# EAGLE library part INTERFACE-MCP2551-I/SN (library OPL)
High speed CAN transceiver
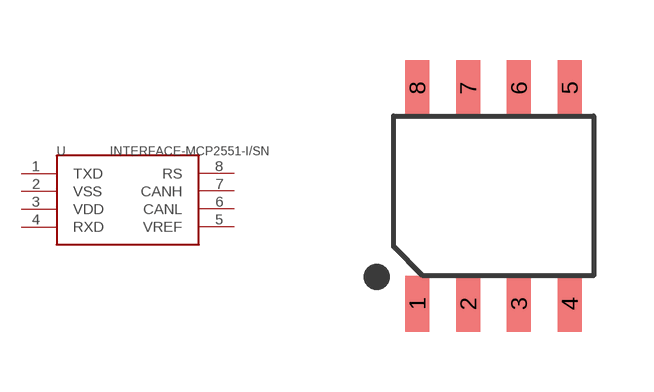
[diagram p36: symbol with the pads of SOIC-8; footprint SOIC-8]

Designator prefix U

## INTERFACE-MCP2551-I/SN-310070024  [SOIC-8]
1  TXD
2  VSS
3  VDD
4  RXD
5  VREF
6  CANL
7  CANH
8  RS

## Footprint SOIC-8 (pad centres in mm)
smd 0.6 x 1.4: 1 -1.905,-2.7; 2 -0.635,-2.7; 3 0.635,-2.7; 4 1.905,-2.7; 5 1.905,2.7; 6 0.635,2.7; 7 -0.635,2.7; 8 -1.905,2.7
